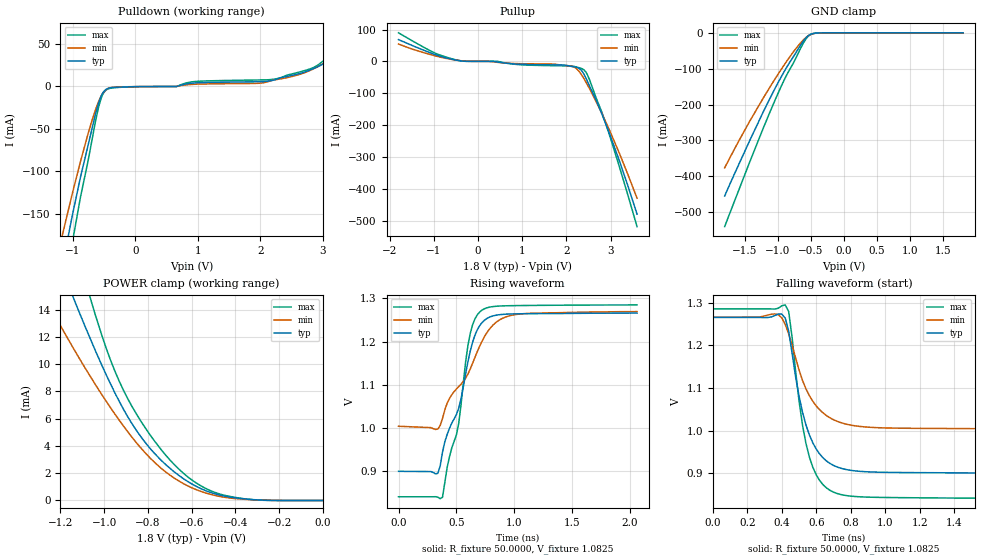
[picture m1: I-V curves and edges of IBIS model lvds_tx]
| Texas Instruments Incorporated
| ADS5294 Octal Channel 14-Bit, 80MSPS High-SNR and Low-Power ADC
| Marketing part#   Voltage Range   Package-type   #pins/pkg drawing
| ADS5294IPFP   1.7V - 1.9V   HTQFP   80/PFP
| ADS5294IPFPR   1.7V - 1.9V   HTQFP   80/PFP
| ADS5294IPFPT   1.7V - 1.9V   HTQFP   80/PFP
[IBIS ver] 3.2
[File name] ads5294.ibs
[File Rev] 1.0
[Date] Mon Nov 16 17:09:14 IST 2009
[Source]   TIspice3 simulations
   Texas Instruments Incorporated.
   Analog eLab Design Center, HPA
   12500 TI Blvd
   Dallas, TX -75243
   For Support e-mail: elab_scm_ibis@list.ti.com
[Disclaimer]  Please be aware that in the absence of a written agreement,
   Texas Instruments (TI) assumes no liability for: 1)
   the accuracy of the IBIS models provided to your company, 2)
   the proper functioning of these IBIS models in your design or
   for any resulting applications, or; 3) infringement of patents,
   copyrights, or intellectual property rights resulting from
   your use of these IBIS models. TI provides IBIS models as a
   service to our customers and therefore reserves the right to
   limit distribution of the IBIS models.
[Copyright] (C)Copyright 2011 Texas Instruments Incorporated.
   All rights reserved.
|   Component ADS529xIPFP
[Component] ADS529xIPFP
[Manufacturer] Texas Instruments.
[Package]
| variable   typ   min   max
R_pkg   0.3702   0.1484   0.5035
L_pkg   3.6148nH   2.8818nH   4.60713nH
C_pkg   0.6034pF   0.5489pF   0.7199pF
[Pin]  signal_name   model_name   R_pin   L_pin   C_pin
 1   TERM   TERM   0.04205  4.38368n  0.42522p
 2   TERM   TERM   0.04186  4.13267n  0.47670p
 3   AVSS   GND   0.04149  3.73032n  0.46954p
 4   TERM   TERM   0.04102  4.02627n  0.46210p
 5   TERM   TERM   0.04052  3.86760n  0.45329p
 6   TERM   TERM   0.03996  3.74206n  0.44390p
 7   TERM   TERM   0.03935  3.72266n  0.43431p
 8   TERM   TERM   0.03879  3.63760n  0.42528p
 9   TERM   TERM   0.03826  3.62612n  0.41727p
10   TERM   TERM   0.03785  3.79229n  0.40794p
11   TERM   TERM   0.03784  3.34817n  0.40797p
12   TERM   TERM   0.03828  3.28983n  0.41721p
13   OUT1A_p   lvds_tx  0.03878  3.69129n  0.42533p
14   OUT1A_n   lvds_tx  0.03936  3.62893n  0.43426p
15   OUT1B_p   lvds_tx  0.03995  3.61722n  0.44395p
16   OUT1B_n   lvds_tx  0.04053  3.60816n  0.45328p
17   OUT2A_p   lvds_tx  0.04101  3.63683n  0.46214p
18   OUT2A_n   lvds_tx  0.04150  3.71171n  0.46954p
19   OUT2B_p   lvds_tx  0.04185  3.81581n  0.47678p
20   OUT2B_p   lvds_tx  0.04206  4.00443n  0.42523p
21   OUT3A_p   lvds_tx  0.04205  3.95118n  0.42523p
22   OUT3A_n   lvds_tx  0.04186  3.69686n  0.47670p
23   OUT3B_p   lvds_tx  0.04149  3.52629n  0.46953p
24   OUT3B_p   lvds_tx  0.04102  3.39247n  0.46210p
25   OUT4A_p   lvds_tx  0.04052  3.56820n  0.45329p
26   OUT4A_n   lvds_tx  0.03996  3.42556n  0.44390p
27   OUT4B_p   lvds_tx  0.03935  3.32916n  0.43431p
28   OUT4B_p   lvds_tx  0.03879  3.26680n  0.42528p
29   ACLK_p   lvds_tx  0.03826  3.34752n  0.41727p
30   ACLK_n   lvds_tx  0.03785  3.28119n  0.40794p
31   LCLK_p   lvds_tx  0.03784  3.25257n  0.40797p
32   LCLK_n   lvds_tx  0.03828  3.25942n  0.41721p
33   OUT5B_p   lvds_tx  0.03878  3.30969n  0.42533p
34   OUT5B_p   lvds_tx  0.03936  3.40523n  0.43426p
35   OUT5A_p   lvds_tx  0.03995  3.47872n  0.44395p
36   OUT5A_n   lvds_tx  0.04053  3.63286n  0.45328p
37   OUT6B_p   lvds_tx  0.04101  3.39613n  0.46214p
38   OUT6B_p   lvds_tx  0.04150  3.53171n  0.46954p
39   OUT6A_p   lvds_tx  0.04185  3.70331n  0.47678p
40   OUT6A_n   lvds_tx  0.04206  3.95903n  0.42523p
41   OUT7B_p   lvds_tx  0.04205  4.11288n  0.42522p
42   OUT7B_p   lvds_tx  0.04186  3.90217n  0.47670p
43   OUT7A_p   lvds_tx  0.04149  3.76449n  0.46953p
44   OUT7A_n   lvds_tx  0.04102  3.66717n  0.46210p
45   OUT8B_p   lvds_tx  0.04052  3.61610n  0.45329p
46   OUT8B_p   lvds_tx  0.03996  3.60246n  0.44390p
47   OUT8A_p   lvds_tx  0.03935  3.62156n  0.43431p
48   OUT8A_n   lvds_tx  0.03879  3.67920n  0.42528p
49   TERM   TERM   0.03826  3.73252n  0.41727p
50   TERM   TERM   0.03785  3.39532n  0.40794p
51   TERM   TERM   0.03784  3.93767n  0.40797p
52   TERM   TERM   0.03828  3.71102n  0.41721p
53   TERM   TERM   0.03878  3.71509n  0.42533p
54   TERM   TERM   0.03936  3.82703n  0.43426p
55   TERM   TERM   0.03995  3.83112n  0.44395p
56   TERM   TERM   0.04053  3.97476n  0.45328p
57   TERM   TERM   0.04101  4.14843n  0.46214p
58   TERM   TERM   0.04150  4.12781n  0.46954p
59   TERM   TERM   0.04185  4.33791n  0.47678p
60   TERM   TERM   0.04206  4.60713n  0.42523p
61   TERM   TERM   0.04205  3.81698n  0.42522p
62   TERM   TERM   0.04186  3.58617n  0.47670p
63   TERM   TERM   0.04149  3.42698n  0.46954p
64   TERM   TERM   0.04102  3.34207n  0.46210p
65   TERM   TERM   0.04052  3.27910n  0.45329p
66   TERM   TERM   0.03996  2.88180n  0.44390p
67   TERM   TERM   0.03935  3.25436n  0.43431p
68   TERM   TERM   0.03879  3.26830n  0.42528p
69   TERM   TERM   0.03826  3.32712n  0.41727p
70   TERM   TERM   0.03785  3.43039n  0.40794p
71   AVDD   POWER   0.03784  3.02476n  0.40797p
72   TERM   TERM   0.03828  3.23992n  0.41721p
73   TERM   TERM   0.03878  3.28049n  0.42533p
74   TERM   TERM   0.03936  2.90922n  0.43426p
75   TERM   TERM   0.03995  3.28952n  0.44395p
76   TERM   TERM   0.04053  3.37086n  0.45328p
77   TERM   TERM   0.04101  3.49703n  0.46214p
78   TERM   TERM   0.04150  3.44761n  0.46954p
79   TERM   TERM   0.04185  3.61371n  0.47678p
80   TERM   TERM   0.04206  3.85493n  0.42523p
[Diff Pin]   inv_pin   vdiff   tdelay_typ   tdelay_min   tdelay_max
   13   14   350mV   0   0   0
   15   16   350mV   0   0   0
   17   18   350mV   0   0   0
   19   20   350mV   0   0   0
   21   22   350mV   0   0   0
   23   24   350mV   0   0   0
   25   26   350mV   0   0   0
   27   28   350mV   0   0   0
   29   30   350mV   0   0   0
   31   32   350mV   0   0   0
   33   34   350mV   0   0   0
   35   36   350mV   0   0   0
   37   38   350mV   0   0   0
   39   40   350mV   0   0   0
   41   42   350mV   0   0   0
   43   44   350mV   0   0   0
   45   46   350mV   0   0   0
   47   48   350mV   0   0   0
[Model]  TERM
Model_type Terminator
C_comp   0   0   0
[Voltage Range]  1.80  1.7  1.9
[Temperature Range] 25   125   -40
| Models and submodels in the file (2): lvds_tx (3-state), TERM (Terminator)
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|   Model lvds_tx
[Model]  lvds_tx
Model_type 3-state
Polarity   Non-Inverting
Enable   Active-Low
Vmeas = 1.065V
Cref = 5.0000pF
Rref = 50.0000
Vref = 1.065V
C_comp   2.2000pF   2.0000pF   2.4000pF
[Temperature Range]   25.0000   0.1250k   -40.0000
[Voltage Range]   1.8000V   1.7000V   1.9000V
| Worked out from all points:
|   slope of the pulldown table from 0 to 0.27 V, typ, clamps not added: 2.11 kohm
|   slope of the pullup table from 0 to 0.27 V, typ, clamps not added: 19.6 kohm
|   GND clamp passes 1 mA (typ) near -0.43 V on its own axis
|   POWER clamp passes 1 mA (typ) near -0.57 V on its own axis
|   rising waveform, R_fixture 50.0000, V_fixture 1.0825: 20-80 % time 228ps typ, 334ps min, 166ps max; typ from 0.899 V to 1.27 V
|   falling waveform, R_fixture 50.0000, V_fixture 1.0825: 20-80 % time 123ps typ, 153ps min, 102ps max; typ from 1.27 V to 0.899 V
[Pulldown]
|Voltage   I(typ)   I(min)   I(max)
-1.8V     -470.2mA   -385.4mA   -558.6mA
-1.19V    -219.2mA   -181mA     -264.4mA
-1.01V    -151.8mA   -126mA     -183.9mA
-880mV    -106.9mA   -88.53mA   -130.3mA
-640mV    -32.81mA   -27.64mA   -41.41mA
-550mV    -11.73mA   -11.48mA   -14.39mA
-450mV    -2.729mA   -2.929mA   -3.419mA
1.96V     5.415mA    3.576mA    7.487mA
2.3V      9.5mA      8.509mA    9.592mA
2.9V      22.47mA    22.43mA    24.06mA
3.29V     40.54mA    39.73mA    44.96mA
3.6V      59.26mA    55.48mA    67.55mA
[Pullup]
|Voltage   I(typ)   I(min)   I(max)
-1.8V     68.69mA    54.82mA    90mA
-990mV    22.5mA     18.4mA     27.38mA
-430mV    2.65mA     3.069mA    2.778mA
2.07V     -14.19mA   -13.88mA   -14.08mA
2.23V     -18.57mA   -22.67mA   -17.47mA
2.33V     -26.46mA   -39.19mA   -21.49mA
2.4V      -40.27mA   -54.59mA   -26.6mA
2.47V     -60.22mA   -71.58mA   -39.92mA
2.53V     -78.99mA   -86.98mA   -59.14mA
2.8V      -163.4mA   -162.4mA   -158.2mA
3.2V      -312.1mA   -288.5mA   -330.8mA
3.6V      -479.7mA   -429.6mA   -518.9mA
[GND_clamp]
|Voltage   I(typ)   I(min)   I(max)
-1.8V     -455.1mA   -376.5mA   -540.2mA
-1.43V    -303.7mA   -249.2mA   -364.1mA
-1.22V    -221.5mA   -182.7mA   -267.1mA
-1.03V    -151.6mA   -125.8mA   -183.6mA
-890mV    -104.4mA   -86.38mA   -127.2mA
-720mV    -54.06mA   -42.92mA   -68.61mA
-610mV    -22.22mA   -19.42mA   -27.81mA
-570mV    -13.4mA    -12.7mA    -16.38mA
-530mV    -7.078mA   -7.493mA   -8.285mA
-460mV    -1.728mA   -2.279mA   -1.919mA
-350mV    -129.4uA   -208.1uA   -178uA
1.8V      2.877nA    325.1nA    670.9pA
[POWER_clamp]
|Voltage   I(typ)   I(min)   I(max)
-1.8V     43.85mA    37.19mA    59.49mA
-1.26V    19.83mA    14.59mA    26.34mA
-1.13V    14.44mA    10.87mA    18.54mA
-1.09V    12.87mA    9.791mA    16.28mA
-1.04V    10.98mA    8.496mA    13.59mA
-950mV    7.865mA    6.317mA    9.449mA
-870mV    5.564mA    4.585mA    6.82mA
-770mV    3.457mA    2.802mA    4.368mA
-620mV    1.416mA    1.09mA     1.761mA
-520mV    624.2uA    477.4uA    765.1uA
-410mV    215.3uA    156.5uA    252.9uA
0V        2.877nA    37.47nA    895.7pA
[Ramp]
| variable   typ   min   max
dV/dt_r  0.7131/0.1616n   0.6999/0.2518n   0.7178/0.1193n
dV/dt_f  0.4975/0.2548n   0.4545/0.4195n   0.5349/0.1799n
R_load = 1.0000k
[Rising Waveform]
R_fixture= 50.0000
V_fixture= 1.0825
V_fixture_min= 1.1350
V_fixture_max= 1.0630
|time   V(typ)   V(min)   V(max)
0s        899mV      1.004V     840mV
340ps     894.4mV    997.3mV    838.9mV
380ps     943.7mV    1.022V     839mV
420ps     984.4mV    1.057V     908mV
520ps     1.045V     1.096V     1.01V
580ps     1.126V     1.115V     1.154V
620ps     1.178V     1.137V     1.219V
720ps     1.244V     1.2V       1.273V
980ps     1.264V     1.261V     1.283V
2.06ns    1.266V     1.269V     1.285V
[Falling Waveform]
R_fixture= 50.0000
V_fixture= 1.0825
V_fixture_min= 1.1350
V_fixture_max= 1.0630
|time   V(typ)   V(min)   V(max)
0s        1.266V     1.267V     1.286V
360ps     1.271V     1.274V     1.286V
420ps     1.265V     1.25V      1.295V
440ps     1.234V     1.227V     1.28V
500ps     1.081V     1.143V     1.07V
560ps     989.8mV    1.082V     937.9mV
620ps     944.7mV    1.049V     882.4mV
700ps     918.2mV    1.026V     855.3mV
980ps     902.1mV    1.007V     842.9mV
2.44ns    899.4mV    1.004V     840mV
